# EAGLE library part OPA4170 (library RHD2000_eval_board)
TI OPA4170 quad op amp
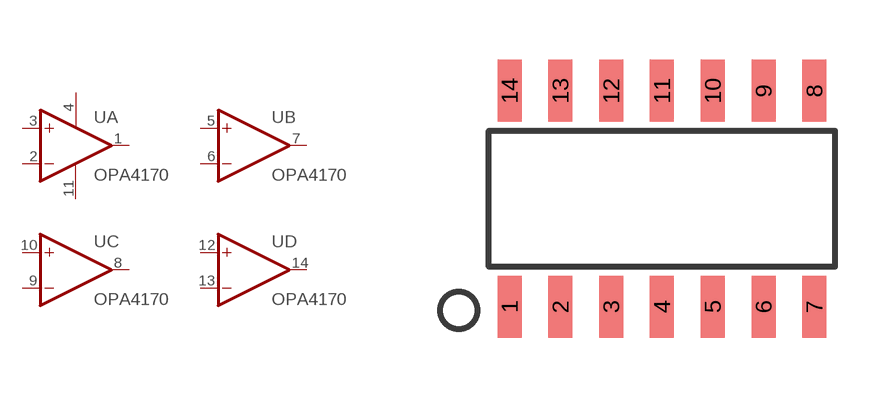
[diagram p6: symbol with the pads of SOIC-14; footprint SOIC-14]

Designator prefix U; gates A=OPAMP B=OPAMP C=OPAMP D=OPAMP P=PWR+-

## OPA4170_SO14  [SOIC-14]
1  A:OUT  out
2  A:-IN  in
3  A:+IN  in
4  P:V+  pwr
5  B:+IN  in
6  B:-IN  in
7  B:OUT  out
8  C:OUT  out
9  C:-IN  in
10  C:+IN  in
11  P:V-  pwr
12  D:+IN  in
13  D:-IN  in
14  D:OUT  out

## Footprint SOIC-14 (pad centres in mm)
smd 0.6 x 1.55: 1 -3.81,-2.7; 2 -2.54,-2.7; 3 -1.27,-2.7; 4 0,-2.7; 5 1.27,-2.7; 6 2.54,-2.7; 7 3.81,-2.7; 8 3.81,2.7; 9 2.54,2.7; 10 1.27,2.7; 11 0,2.7; 12 -1.27,2.7; 13 -2.54,2.7; 14 -3.81,2.7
